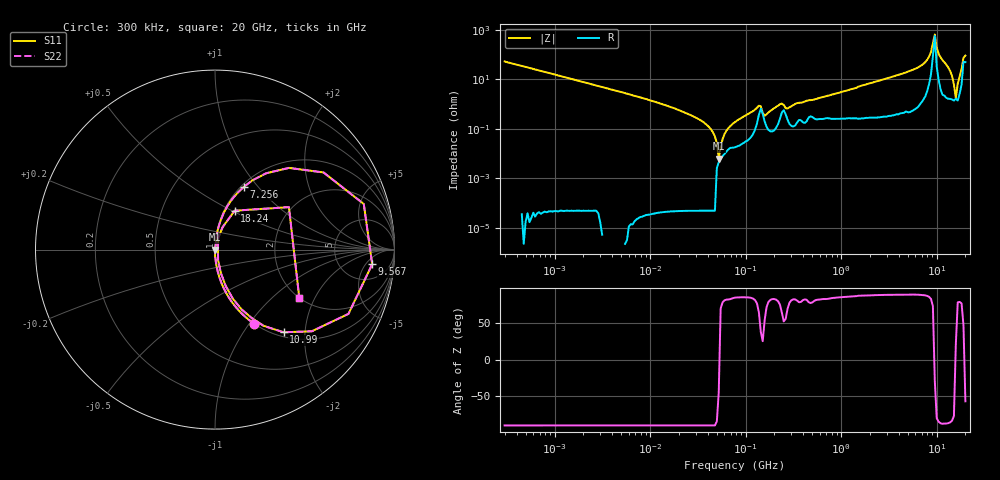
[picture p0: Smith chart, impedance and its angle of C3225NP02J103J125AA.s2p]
! S-parameter Generated by TDK Corporation
! Copyright(C) 2015 TDK Corporation.
! All Rights Reserved.
! TDK P/N: C3225NP02J103J125AA (Multilayer Ceramic Chip Capacitors)
! Property: C=10nF
! Size(LxWxT): 3.2x2.5x1.25mm, 0.126x0.098x0.049inches
! Model Type: s2p (Touchstone File Format Version 1.0)
! Frequency: DC=Yes Start=0.3MHz Stop=20000MHz 243points Log-sweep
! Note:
! Model Generated on Jun. 23, 2015
! Hash(MD5):
! Port Assignments:
!  1 ---| |--- 2
! Applicable Conditions:
!  Temperature = 25 degC
!  DC Bias Voltage = 0 V
!  Small Signal Operation
! Terms and conditions regarding TDK Simulation Models
! (1)This simulation model is being provided solely for informational purposes. Please refer to the specifications of the products in terms of detailed characteristics of such products.
! (2)In no event shall TDK Corporation of any of its subsidiaries be liable for any loss or damage arising, directly or indirectly,
!  From any information contained in this simulation model, including, but not limited to loss or damages arising from any inaccuracies, omissions or errors in connection with such information.
! (3)Any and all copyrights on this simulation model are owned by TDK Corporation.
!  Duplication or redistribution of this simulation model without prior written permission from TDK Corporation is prohibited.
! (4)This simulation model is subject to any modification or change without any prior notice.
! (5)Neither TDK Corporation nor any of its subsidiaries shall make any warranty, express or implied,
!  Including but not limited to the correctness, implied warranties of merchantability and fitness for a particular purpose with respect to this simulation models.
! (6)The use of this simulation model shall be deemed to have consented to the terms and conditions hereof.
# MHz S MA R 50
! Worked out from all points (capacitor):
!   242 points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, 300 kHz to 20 GHz, reference 50 ohm
!   read as one part in series: C = 10.1 nF near 314.2 kHz
!   lowest |Z| = 6.34 mohm at 52.35 MHz (marker M1)
!   series resonance near 52.87 MHz, so ESL is about 900 pH
!   S11 on the Smith chart (normalised r, x): 300 kHz: 1.00, -1.05; 7.256 GHz: 1.03, +0.84; 9.567 GHz: 10, -7; 10.99 GHz: 1.08, -1.55; 18.24 GHz: 1.12, +0.52; 20 GHz: 1.99, -1.53
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0.3  0.4655 -62.3  0.885 27.7  0.885 27.7  0.4655 -62.3
1.985118  0.07855 -85.5  0.9969 4.5  0.9969 4.5  0.07855 -85.5
12.54397  0.01089 -93.0  0.9993 0.6  0.9993 0.6  0.01089 -93.0
37.91615  0.001628 -91.8  0.9999 0.1  0.9999 0.1  0.001628 -91.8
47.74252  0.0004916 -90.0  1 0.0  1 0.0  0.0004916 -90.0
52.35254  6.204e-05 -44.2  1 0.0  1 0.0  6.204e-05 -44.2
60.11549  0.0006206 80.9  0.9999 -0.0  0.9999 -0.0  0.0006206 80.9
79.26541  0.002028 84.6  0.9998 -0.1  0.9998 -0.1  0.002028 84.6
137.8092  0.008609 63.9  0.9962 -0.4  0.9962 -0.4  0.008609 63.9
158.2439  0.003419 53.5  0.998 -0.2  0.998 -0.2  0.003419 53.5
239.5924  0.01057 63.6  0.9953 -0.5  0.9953 -0.5  0.01057 63.6
500.8786  0.0147 77.3  0.9969 -0.8  0.9969 -0.8  0.0147 77.3
3165.055  0.1147 81.8  0.9901 -6.6  0.9901 -6.6  0.1147 81.8
7255.597  0.3829 65.5  0.9101 -22.5  0.9101 -22.5  0.3829 65.5
8724.45  0.7418 35.4  0.5831 -47.4  0.5831 -47.4  0.7418 35.4
9566.884  0.8796 -5.3  0.1353 23.8  0.1353 23.8  0.8796 -5.3
10985.48  0.5982 -50.3  0.7699 36.7  0.7699 36.7  0.5982 -50.3
13832.49  0.2123 -73.5  0.9616 12.2  0.9616 12.2  0.2123 -73.5
15883.6  0.01796 23.8  0.9836 -0.3  0.9836 -0.3  0.01796 23.8
18238.85  0.243 63.2  0.9147 -13.7  0.9147 -13.7  0.243 63.2
19099.14  0.4749 29.9  0.6172 -17.9  0.6172 -17.9  0.4749 29.9
20000  0.5425 -30.0  0.5954 27.1  0.5954 27.1  0.5425 -30.0
